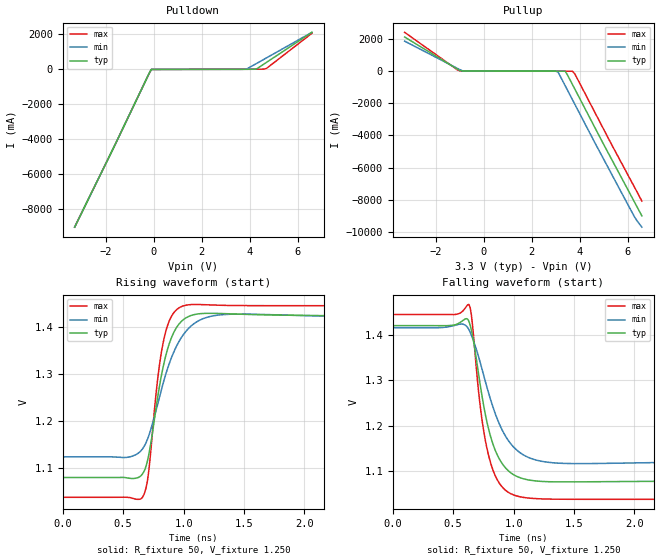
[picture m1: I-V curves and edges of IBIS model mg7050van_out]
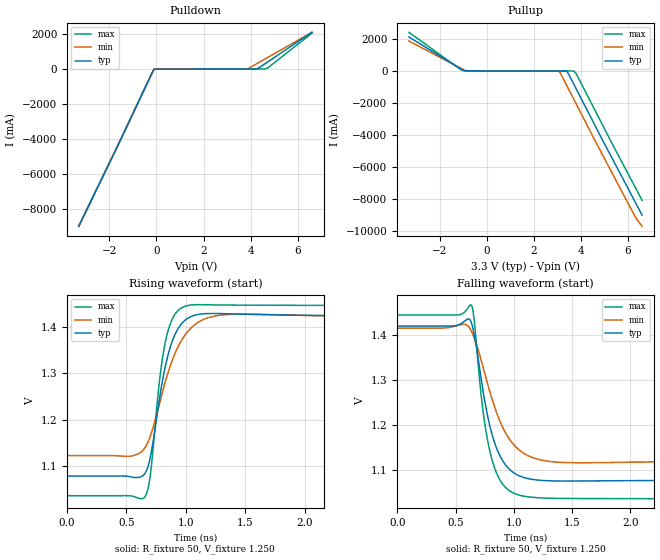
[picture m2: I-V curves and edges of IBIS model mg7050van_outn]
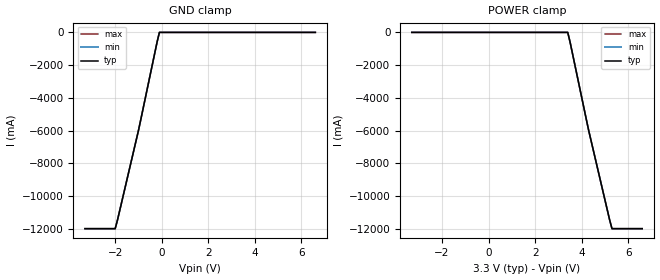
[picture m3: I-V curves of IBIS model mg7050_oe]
|   IBIS File mg7050van_4out_33v.ibs
[IBIS Ver]   3.2
[Comment Char]   |_char
[File name]   mg7050van_4out_33v.ibs
[File Rev]   1.0
[Date]   Aug 02, 2013
[Source]
|   Component MG7050VAN LVDS 4-OUTPUT 3.3V
[Component]   mg7050van-lvds-4out
[Manufacturer]   Seiko Epson Corporation
[Package]
| variable   typ   min   max
R_pkg   0.27   NA   NA
L_pkg   1.66n   NA   NA
C_pkg   0.53p   NA   NA
[Pin]   signal_name   model_name   R_pin   L_pin   C_pin
1   vcc1   POWER   NA   NA   NA
2   out1p   mg7050van_out   0.34   2.1nH   0.58pF
3   out1n   mg7050van_outn  0.25   1.5nH   0.50pF
4   out2p   mg7050van_out   0.22   1.3nH   0.44pF
5   out2n   mg7050van_outn  0.25   1.7nH   0.59pF
6   fsel   mg7050_fsel   NA   NA   NA
7   oe   mg7050_oe   NA   NA   NA
8   out3n   mg7050van_outn  0.25   1.7nH   0.62pF
9   out3p   mg7050van_out   0.22   1.3nH   0.49pF
10   out4n   mg7050van_outn  0.25   1.5nH   0.46pF
11   out4p   mg7050van_out   0.34   2.1nH   0.57pF
12   vcc2   POWER   NA   NA   NA
13   vcc   POWER   NA   NA   NA
14   gnd   GND   NA   NA   NA
[Diff Pin] inv_pin vdiff   tdelay_typ
2   3   0   0
4   5   0   0
9   8   0   0
11   10   0   0
| Models and submodels in the file (4): mg7050van_out (Output), mg7050van_outn (Output), mg7050_oe (Input), mg7050_fsel (Input)
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[Model]   mg7050van_out
Model_type Output
Enable Active-High
Polarity Non-Inverting
Vref=1.250
Vmeas=1.250
Rref=50
Cref=0
C_comp   0.12p   0.12p   0.12p
[Temperature Range] 25   90   -40
[Voltage Range]   3.3   2.97   3.63
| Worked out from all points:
|   slope of the pulldown table from 0 to 0.495 V, typ, clamps not added: 254 ohm
|   slope of the pullup table from 0 to 0.495 V, typ, clamps not added: 184 ohm
|   falling waveform, R_fixture 50, V_fixture 1.250: 20-80 % time 159ps typ, 221ps min, 129ps max; typ from 1.42 V to 1.08 V
|   rising waveform, R_fixture 50, V_fixture 1.250: 20-80 % time 143ps typ, 214ps min, 106ps max; typ from 1.08 V to 1.42 V
[Pullup]
-3.3V     2.123A     1.868A     2.416A
-1.1V     125.6mA    171.3mA    81.55mA
-1V       38.39mA    94.22mA    18.59mA
-800mV    8.375mA    7.832mA    11.52mA
3V        -3.675mA   -3.087mA   -4.521mA
3.1V      -3.683mA   -53.21mA   -4.552mA
3.4V      -3.704mA   -910.8mA   -4.609mA
3.7V      -825.1mA   -1.77A     -4.642mA
3.8V      -1.112A    -2.057A    -166.5mA
5.3V      -5.383A    -6.305A    -4.464A
6.3V      -8.175A    -9.094A    -7.248A
6.6V      -9.012A    -9.711A    -8.09A
[Pulldown]
-3.3V     -9.013A    -9.012A    -9.015A
-1.7V     -4.547A    -4.546A    -4.548A
-200mV    -251.2mA   -251mA     -251.3mA
-100mV    -851.5uA   -637uA     -1.086mA
3.8V      7.885mA    11mA       9.866mA
3.9V      8.474mA    42.2mA     10.37mA
4.3V      39.33mA    348.4mA    13.84mA
4.6V      307.7mA    579.1mA    18.51mA
4.7V      398.4mA    656mA      53.33mA
6.6V      2.121A     2.118A     2.066A
[Falling Waveform]
R_fixture=50
V_fixture=1.250
V_fixture_min=1.271
V_fixture_max=1.238
0s        1.42V      1.416V     1.445V
520ps     1.422V     1.421V     1.445V
630ps     1.43V      1.412V     1.467V
660ps     1.398V     1.393V     1.422V
730ps     1.279V     1.333V     1.23V
790ps     1.196V     1.275V     1.138V
880ps     1.128V     1.205V     1.074V
1ns       1.092V     1.153V     1.048V
1.4ns     1.076V     1.117V     1.038V
4ns       1.078V     1.122V     1.038V
[Rising Waveform]
R_fixture=50
V_fixture=1.250
V_fixture_min=1.271
V_fixture_max=1.238
0s        1.079V     1.123V     1.037V
660ps     1.087V     1.14V      1.037V
710ps     1.126V     1.167V     1.09V
780ps     1.241V     1.23V      1.277V
830ps     1.314V     1.279V     1.365V
900ps     1.377V     1.335V     1.423V
990ps     1.414V     1.381V     1.444V
1.14ns    1.428V     1.415V     1.448V
1.36ns    1.428V     1.427V     1.446V
4ns       1.423V     1.419V     1.445V
[Ramp]
R_load=50
dV/dt_r   2.063E-1/1.433E-10   1.773E-1/2.136E-10   2.449E-1/1.064E-10
dV/dt_f   2.055E-1/1.587E-10   1.762E-1/2.205E-10   2.441E-1/1.289E-10
|[End   mg7050van_out
[Model]   mg7050van_outn
Model_type Output
Enable Active-High
Polarity Inverting
Vref=1.250
Vmeas=1.250
Rref=50
Cref=0
C_comp   0.12p   0.12p   0.12p
[Temperature Range] 25   90   -40
[Voltage Range]   3.3   2.97   3.63
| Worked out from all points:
|   slope of the pulldown table from 0 to 0.495 V, typ, clamps not added: 254 ohm
|   slope of the pullup table from 0 to 0.495 V, typ, clamps not added: 184 ohm
|   falling waveform, R_fixture 50, V_fixture 1.250: 20-80 % time 165ps typ, 229ps min, 134ps max; typ from 1.42 V to 1.08 V
|   rising waveform, R_fixture 50, V_fixture 1.250: 20-80 % time 146ps typ, 218ps min, 108ps max; typ from 1.08 V to 1.42 V
[Pullup]
-3.3V     2.122A     1.867A     2.415A
-1.1V     125.5mA    171.2mA    81.51mA
-1V       38.38mA    94.19mA    18.59mA
-800mV    8.375mA    7.832mA    11.52mA
3V        -3.675mA   -3.087mA   -4.521mA
3.1V      -3.683mA   -53.21mA   -4.552mA
3.4V      -3.704mA   -910.8mA   -4.609mA
3.7V      -825.1mA   -1.77A     -4.642mA
3.8V      -1.112A    -2.057A    -166.5mA
5.3V      -5.383A    -6.305A    -4.464A
6.3V      -8.175A    -9.094A    -7.248A
6.6V      -9.012A    -9.711A    -8.09A
[Pulldown]
-3.3V     -9.013A    -9.012A    -9.015A
-1.7V     -4.547A    -4.546A    -4.548A
-200mV    -251.2mA   -251mA     -251.3mA
-100mV    -851.5uA   -637uA     -1.086mA
3.8V      7.885mA    11mA       9.866mA
3.9V      8.474mA    42.19mA    10.37mA
4.3V      39.32mA    348.3mA    13.84mA
4.6V      307.6mA    579mA      18.51mA
4.7V      398.2mA    655.9mA    53.31mA
6.6V      2.121A     2.118A     2.066A
[Falling Waveform]
R_fixture=50
V_fixture=1.250
V_fixture_min=1.271
V_fixture_max=1.238
0s        1.42V      1.416V     1.445V
580ps     1.432V     1.424V     1.452V
640ps     1.424V     1.407V     1.465V
660ps     1.401V     1.394V     1.433V
730ps     1.286V     1.335V     1.243V
800ps     1.192V     1.269V     1.137V
890ps     1.128V     1.204V     1.075V
1.02ns    1.091V     1.151V     1.047V
1.42ns    1.076V     1.118V     1.038V
4ns       1.078V     1.122V     1.037V
[Rising Waveform]
R_fixture=50
V_fixture=1.250
V_fixture_min=1.271
V_fixture_max=1.238
0s        1.079V     1.123V     1.037V
520ps     1.079V     1.122V     1.037V
660ps     1.087V     1.142V     1.037V
700ps     1.118V     1.164V     1.079V
780ps     1.248V     1.236V     1.287V
830ps     1.318V     1.284V     1.37V
900ps     1.378V     1.337V     1.423V
990ps     1.413V     1.381V     1.443V
1.36ns    1.428V     1.426V     1.446V
4ns       1.423V     1.419V     1.446V
[Ramp]
R_load=50
dV/dt_r   2.064E-1/1.457E-10   1.772E-1/2.178E-10   2.449E-1/1.080E-10
dV/dt_f   2.054E-1/1.646E-10   1.761E-1/2.286E-10   2.443E-1/1.336E-10
|[End   mg7050van_outn
[Model]   mg7050_oe
Model_type Input
Vinh=2.31
Vinl=0.99
C_comp   3p   3p   3p
[Temperature Range] 25   90   -40
[Voltage Range]   3.3   2.97   3.63
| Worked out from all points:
|   GND clamp passes 1 mA (typ) near -0.10 V on its own axis
[GND Clamp]
-3.3V     -12A       -12A       -12A
-2V       -12A       -12A       -12A
-1.9V     -11.47A    -11.47A    -11.47A
-1V       -6A        -6A        -6A
-200mV    -592.5mA   -592.5mA   -592.5mA
-100mV    -33.15uA   -27.83uA   -40.33uA
6.6V      32.19uA    32.97uA    32.12uA
[POWER Clamp]
-3.3V     32.19uA    32.97uA    32.12uA
3.4V      -33.15uA   -27.83uA   -40.33uA
3.5V      -592.5mA   -592.5mA   -592.5mA
4.3V      -6A        -6A        -6A
5.2V      -11.47A    -11.47A    -11.47A
5.3V      -12A       -12A       -12A
6.6V      -12A       -12A       -12A
